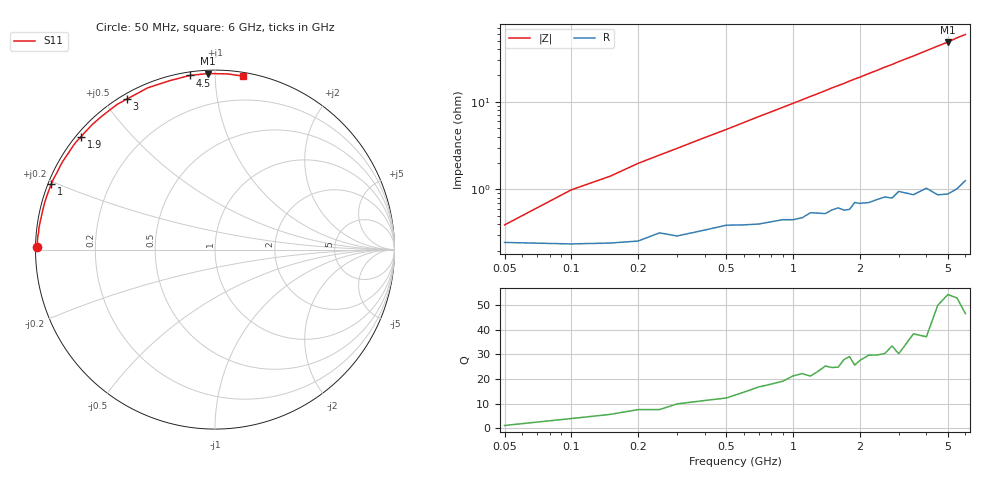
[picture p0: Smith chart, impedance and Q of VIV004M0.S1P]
! Infineon Technologies  Discrete & RF Semiconductors
! BB 804
! Si Tuning Diode in SOT23
! VR =
! S-Parameters:  July  1999
# GHz  S  MA  R  50
!  f  S11
! GHz  MAG  ANG
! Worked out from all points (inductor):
!   34 points, 50 MHz to 6 GHz, reference 50 ohm
!   read as one part to ground: L = 1.53 nH near 100 MHz
!   highest Q = 52.8 at 5 GHz (marker M1), where L = 1.53 nH
!   S11 on the Smith chart (normalised r, x): 50 MHz: 0.00, +0.01; 1 GHz: 0.01, +0.19; 1.9 GHz: 0.01, +0.36; 3 GHz: 0.02, +0.57; 4.5 GHz: 0.02, +0.86; 6 GHz: 0.03, +1.17
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0.05  0.9901 179.3
0.1  0.9905 177.8
0.15  0.9903 176.8
0.2  0.9898 175.5
0.25  0.9873 174.4
0.3  0.9883 173.3
0.6  0.9846 166.8
0.8  0.9834 162.5
1  0.9828 158.3
1.1  0.982 156.2
1.4  0.9804 150.0
1.5  0.9787 147.9
1.6  0.9777 146.0
1.7  0.9792 144.1
1.8  0.979 142.0
1.9  0.9753 140.0
2  0.9761 138.3
2.2  0.9762 134.4
2.4  0.9749 130.9
2.6  0.9741 127.1
2.8  0.9755 123.9
3  0.9718 120.3
3.5  0.9762 112.6
4  0.9743 105.1
4.5  0.9803 98.3
5  0.9817 92.3
5.5  0.9813 85.9
6  0.979 80.9
